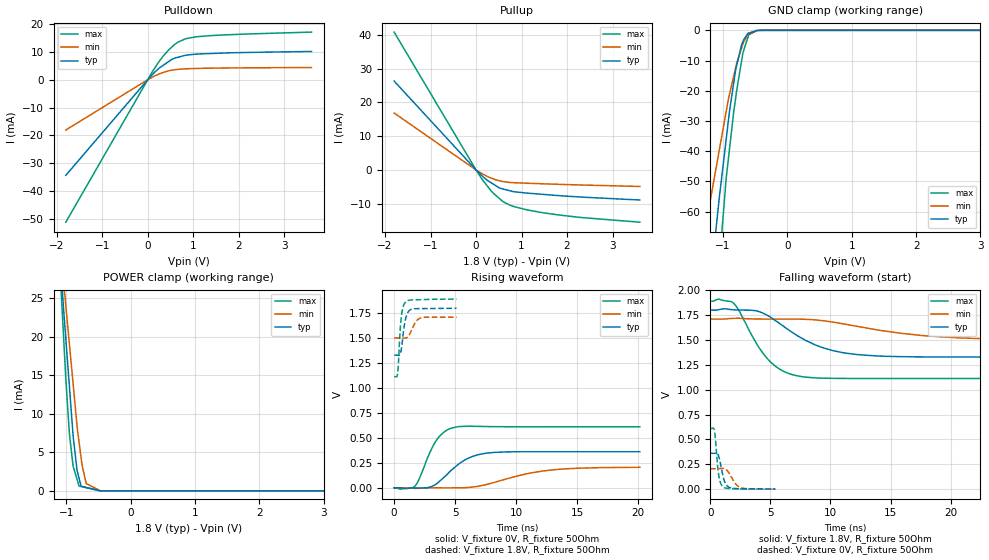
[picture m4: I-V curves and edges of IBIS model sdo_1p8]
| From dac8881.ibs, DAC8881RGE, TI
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|   sdo_1p8 Model
[Model]   sdo_1p8
Model_type   3-state
Polarity   Non-Inverting
Vmeas = 0.9
Vref = 0.9
Cref = 50pF
Rref = 50
|   typ   min   max
|   (nom PVT)   (fast PVT)   (slow PVT)
|C_comp from frequency sweep method (F=25MHz)
C_comp   6.052e-12   5.178e-12   7.110e-12
|ON state : BUFFER OUTPUT TURNED HIGH
|C_comp   6.052e-12   5.178e-12   7.110e-12
|OFF state: BUFFER IN HIGH IMPEDANCE
|C_comp   4.138e-12   3.224e-12   4.977e-12
|C_comp from LC tank measurement(L=1nH)
|Resonant Frequency(Hz)   2.800e+09   3.070e+09   2.590e+09
|C_comp   3.234e-12   2.690e-12   3.780e-12
|ON state : BUFFER OUTPUT TURNED HIGH
|Resonant Frequency(Hz)   2.800e+09   3.070e+09   2.590e+09
|C_comp   3.234e-12   2.690e-12   3.780e-12
|OFF state: BUFFER IN HIGH IMPEDANCE
|Resonant Frequency(Hz)   2.820e+09   3.110e+09   2.590e+09
|C_comp   3.188e-12   2.622e-12   3.780e-12
| Where nom  PVT is Nominal Process, 1.8V, 25C
|   Fast PVT is Strong Process,  1.89V, -40C
|   Slow PVT is Weak Process,   1.71V, 105C
[Voltage Range]   1.8   1.71   1.89
|Ambient Temperature   25   105   -40
|Junction Temperature
[Temperature Range]   25   105   -40
[Pullup Reference]   1.8   1.71   1.89
[Pulldown Reference]   0   0   0
[Power Clamp Reference]   1.8   1.71   1.89
[GND Clamp Reference]   0   0   0
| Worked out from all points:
|   slope of the pulldown table from 0 to 0.27 V, typ, clamps not added: 61.4 ohm
|   slope of the pullup table from 0 to 0.27 V, typ, clamps not added: 82.6 ohm
|   GND clamp passes 1 mA (typ) near -0.62 V on its own axis
|   POWER clamp passes 1 mA (typ) near -0.78 V on its own axis
|   falling waveform, V_fixture 1.8V, R_fixture 50Ohm: 20-80 % time 4.06ns typ, 7.08ns min, 2.44ns max; typ from 1.8 V to 1.33 V
|   rising waveform, V_fixture 0V, R_fixture 50Ohm: 20-80 % time 2.18ns typ, 4.17ns min, 1.37ns max; typ from 0 V to 0.361 V
|   rising waveform, V_fixture 1.8V, R_fixture 50Ohm: 20-80 % time 334ps typ, 513ps min, 252ps max; typ from 1.33 V to 1.8 V
|   falling waveform, V_fixture 0V, R_fixture 50Ohm: 20-80 % time 413ps typ, 650ps min, 288ps max; typ from 0.361 V to 0.001 V
[Pulldown]
|   Voltage   I(typ)   I(min)   I(max)
-1.8V     -34.4mA    -18.09mA   -51.27mA
107.7mV   1.937mA    991.6uA    3.036mA
252mV     4.192mA    2.061mA    6.588mA
332.6mV   5.107mA    2.58mA     8.353mA
451.7mV   6.457mA    3.16mA     10.59mA
574.6mV   7.635mA    3.573mA    12.46mA
667.2mV   8.107mA    3.73mA     13.56mA
835.4mV   8.812mA    3.936mA    14.78mA
1.089V    9.234mA    4.075mA    15.5mA
1.784V    9.681mA    4.243mA    16.21mA
3.6V      10.18mA    4.405mA    17.16mA
[GND Clamp]
|   Voltage   I(typ)   I(min)   I(max)
-1.8V     -217mA     -139.8mA   -308mA
-1.274V   -99.43mA   -65.22mA   -142.1mA
-1.26V    -96.33mA   -63.56mA   -137.7mA
-1.217V   -87.61mA   -58.47mA   -124.2mA
-1.058V   -55.34mA   -39.59mA   -77.1mA
-952.6mV  -36.24mA   -27mA      -49.27mA
-898.2mV  -26.49mA   -21.01mA   -38.92mA
-802.8mV  -12.87mA   -12.22mA   -22.15mA
-691.7mV  -3.725mA   -4.522mA   -7.539mA
-615.6mV  -1.003mA   -1.392mA   -2.43mA
-447.9mV  -20.36uA   -41.93uA   -17.08uA
3.6V      0A         0A         0A
[Pullup]
|   Voltage   I(typ)   I(min)   I(max)
-1.8V     26.3mA     16.84mA    40.8mA
0V        0A         0A         0A
139.9mV   -1.835mA   -1.15mA    -2.9mA
332.6mV   -3.8mA     -2.396mA   -6.214mA
495mV     -5.179mA   -3.159mA   -8.234mA
574.6mV   -5.586mA   -3.409mA   -9.177mA
825.9mV   -6.427mA   -3.77mA    -10.82mA
1.542V    -7.309mA   -4.136mA   -12.81mA
2.362V    -8.066mA   -4.472mA   -14.14mA
3.6V      -8.89mA    -4.89mA    -15.46mA
[POWER Clamp]
|   Voltage   I(typ)   I(min)   I(max)
-1.8V     120.2mA    102.8mA    142.5mA
-1.077V   27.95mA    30.13mA    25.25mA
-1.048V   24.02mA    27.48mA    20.6mA
-1.007V   19.55mA    23.88mA    14.32mA
-952.6mV  13.47mA    18.98mA    7.376mA
-892.8mV  6.906mA    13.64mA    3.122mA
-833.4mV  2.627mA    8.336mA    1.469mA
-803.3mV  1.637mA    6.338mA    630.3uA
-757.5mV  588.1uA    3.388mA    543.7uA
-692.5mV  454.4uA    965.6uA    420.6uA
-470.3mV  32.81nA    1.628uA    0A
3.6V      0A         0A         0A
[Ramp]
R_load = 50
|   typ   min   max
dV/dt_r   0.216668/2.1757e-09   0.123608/4.16925e-09   0.366666/1.37482e-09
dV/dt_f   0.283328/4.05944e-09   0.125809/7.06281e-09   0.466188/2.44616e-09
[Falling Waveform]
V_fixture = 1.8V
V_fixture_min = 1.71V
V_fixture_max = 1.89V
R_fixture = 50Ohm
|   Time   V(typ)   V(min)   V(max)
0s        1.8V       1.71V      1.89V
1.904ns   1.803V     1.717V     1.874V
4.008ns   1.787V     1.71V      1.432V
4.84ns    1.741V     1.71V      1.3V
6.064ns   1.64V      1.71V      1.187V
7.584ns   1.519V     1.709V     1.132V
10.25ns   1.392V     1.679V     1.114V
13.84ns   1.339V     1.602V     1.113V
20.78ns   1.328V     1.52V      1.113V
37ns      1.328V     1.5V       1.113V
[Rising Waveform]
V_fixture = 0V
V_fixture_min = 0V
V_fixture_max = 0V
R_fixture = 50Ohm
|   Time   V(typ)   V(min)   V(max)
0s        736.5pV    989.5pV    609.4pV
1.696ns   -1.764mV   -5.98mV    16.16mV
2.064ns   -1.89mV    -4.376mV   90.34mV
3.4ns     33.69mV    -685.8uV   463mV
3.896ns   83.09mV    -805.8uV   537.4mV
4.656ns   172.1mV    -866.7uV   595.6mV
6.144ns   299.3mV    3.882mV    616.5mV
7.6ns     347.1mV    33.43mV    613.2mV
13ns      361.1mV    179.3mV    611.1mV
20.15ns   361.1mV    205.1mV    611.1mV
[Rising Waveform]
V_fixture = 1.8V
V_fixture_min = 1.71V
V_fixture_max = 1.89V
R_fixture = 50Ohm
|   Time   V(typ)   V(min)   V(max)
0s        1.328V     1.5V       1.113V
264ps     1.328V     1.5V       1.128V
328ps     1.327V     1.5V       1.203V
480ps     1.335V     1.5V       1.552V
568ps     1.374V     1.5V       1.688V
704ps     1.496V     1.5V       1.797V
896ps     1.668V     1.498V     1.855V
1.28ns    1.779V     1.541V     1.879V
2.16ns    1.794V     1.7V       1.884V
5.12ns    1.798V     1.708V     1.89V
[Falling Waveform]
V_fixture = 0V
V_fixture_min = 0V
V_fixture_max = 0V
R_fixture = 50Ohm
|   Time   V(typ)   V(min)   V(max)
0s        361.1mV    206mV      611.1mV
328ps     360.9mV    205.9mV    601.6mV
408ps     361.9mV    205.8mV    537mV
704ps     331.6mV    205.9mV    143.4mV
1.032ns   149.2mV    208.5mV    27.03mV
1.216ns   70.9mV     205.1mV    13.17mV
1.472ns   25.74mV    178.4mV    7.646mV
2.072ns   6.48mV     60.02mV    4.757mV
2.552ns   4.793mV    14.41mV    2.853mV
5.408ns   1.288mV    1.983mV    218.5uV
